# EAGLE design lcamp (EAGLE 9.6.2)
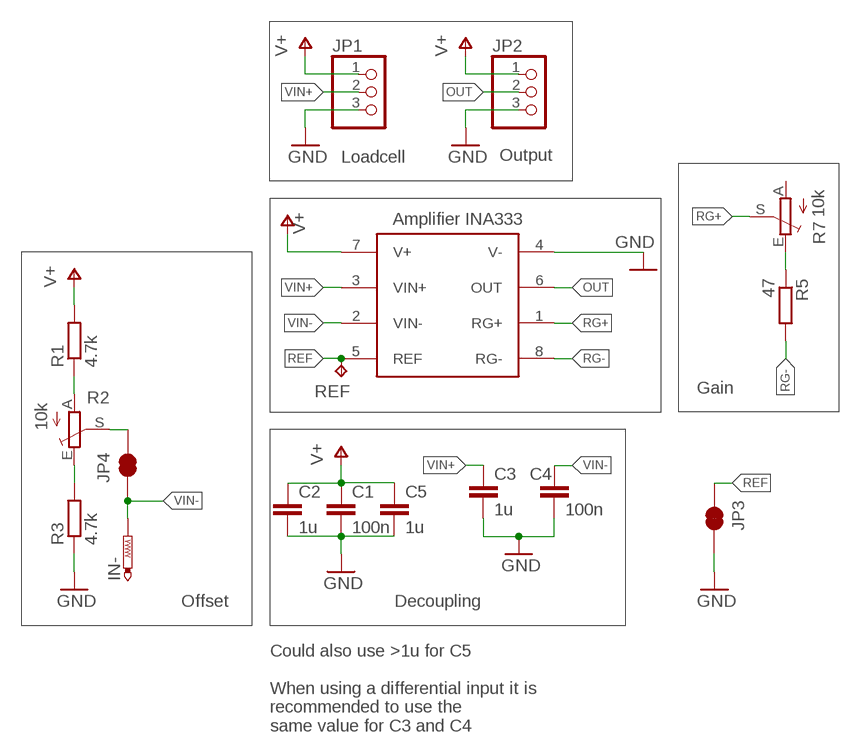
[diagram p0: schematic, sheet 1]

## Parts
C1  100n  C-EUC0603  [C0603]
C2  1u  C-EUC0603  [C0603]
C3  1u  C-EUC0603  [C0603]
C4  100n  C-EUC0603  [C0603]
C5  1u  C-EUC0603  [C0603]
IN-  PTR1PAD1-13  [P1-13]
JP1  PINHD-1X3  [1X03]
JP2  PINHD-1X3  [1X03]
JP3  JUMPER-SMT_2_NC_TRACE_SILK  [SMT-JUMPER_2_NC_TRACE_SILK]
JP4  JUMPER-SMT_2_NC_TRACE_SILK  [SMT-JUMPER_2_NC_TRACE_SILK]
R1  4.7k  R-EU_R0603  [R0603]
R2  10k  TRIM_EU-RJ9W  [RJ9W]
R3  4.7k  R-EU_R0603  [R0603]
R5  47  R-EU_R0603  [R0603]
R7  10k  TRIM_EU-RJ9W  [RJ9W]
REF  TPB1,27  [B1,27]
U1  INA333MSOP8  [MSOP8]

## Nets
GND: C1.2 C2.2 C3.2 C4.2 C5.2 JP1.3 JP2.3 JP3.2 R3.1 U1.4(V-)
N$1: R5.1 R7.E
N$2: R1.1 R2.A
N$3: R2.E R3.2
N$4: JP4.2 R2.S
OUT: JP2.2 U1.6(OUT)
REF: JP3.1 REF.TP U1.5(REF)
RG+: R7.S U1.1(RG+)
RG-: R5.2 U1.8(RG-)
V+: C1.1 C2.1 C5.1 JP1.1 JP2.1 R1.2 U1.7(V+)
VIN+: C3.1 JP1.2 U1.3(VIN+)
VIN-: C4.1 IN-.TP JP4.1 U1.2(VIN-)
Unconnected: R7.A

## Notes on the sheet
- Loadcell | Output
- Amplifier INA333
- Gain
- Offset | Decoupling
- Could also use >1u for C5
  
  When using a differential input it is
  recommended to use the 
  same value for C3 and C4

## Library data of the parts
C1-C5 = resistor:C-EU: CAPACITOR, European symbol
IN- = testpad:PTR1: TEST PIN
JP1 JP2 = pinhead:PINHD-1X3: PIN HEADER
JP3 JP4 = SparkFun-Jumpers:JUMPER-SMT_2_NC_TRACE: Normally closed trace jumper
R1 R3 R5 = resistor:R-EU_: RESISTOR, European symbol
R2 R7 = pot:TRIM_EU-: POTENTIOMETER
REF = testpad:TP: Test pad
U1 = lcamp:INA333

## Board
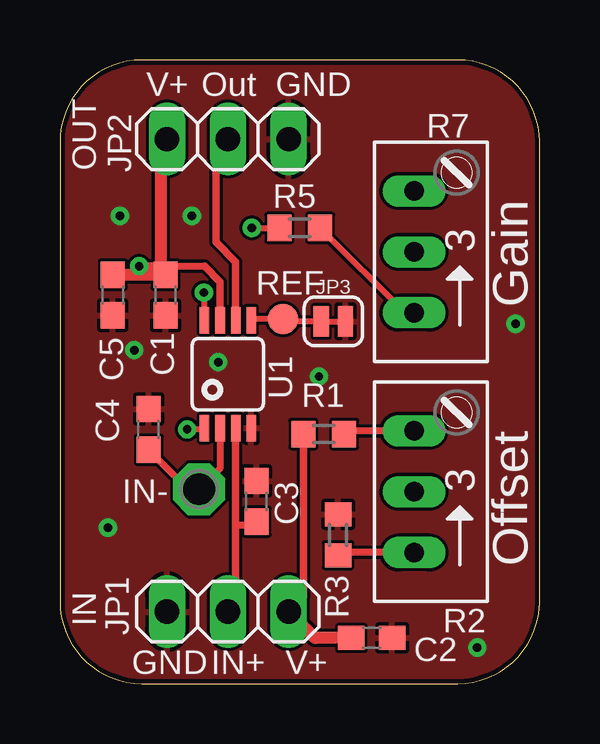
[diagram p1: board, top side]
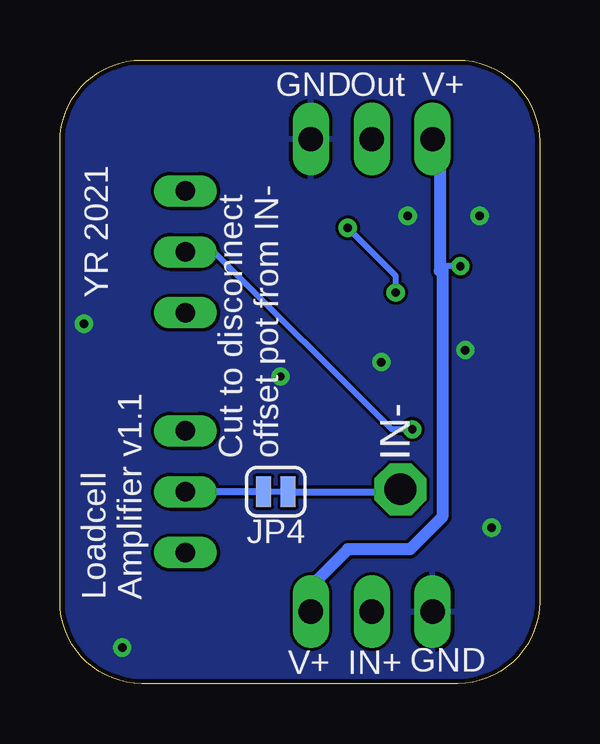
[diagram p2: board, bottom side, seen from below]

Size 20 x 26 mm. Coordinates in mm from the lower left corner, seen from the top.
Outline: 0,22.59 0,3.41 arc90 3.41,0 16.59,0 arc90 20,3.41 20,22.59 arc90 16.59,26 3.41,26 arc90 0,22.59
Copper layers (1*16): Top 0.035mm / dielectric 1.5mm / Bottom 0.035mm
Design rules "jlcpcb": minimum track width 5mil, minimum drill 0.3mm, track to track 5mil, track to pad 5mil, pad to pad 5mil, via to via 5mil, smd to smd 5mil, copper to edge 0.2mm, drill to drill 8mil, minimum pad ring 10mil, minimum via ring 8mil, stop-mask expansion 4mil, vias tented up to drill 0mil, thermal gap 6mil

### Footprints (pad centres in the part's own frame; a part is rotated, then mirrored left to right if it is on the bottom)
C0603 = smd 1.1 x 1: 1 -0.85,0; 2 0.85,0
P1-13 = drill 1.321 pad 2.159 octagon: TP 0,0
1X03 = drill 1.016 long: 1 -2.54,0; 2 0,0; 3 2.54,0
SMT-JUMPER_2_NC_TRACE_SILK = smd 0.635 x 1.27: 1 -0.508,0; 2 0.508,0
R0603 = smd 1 x 1.1: 1 -0.85,0; 2 0.85,0
RJ9W = drill 0.813 long: A 2.54,0.635; E -2.54,0.635; S 0,0.635
B1,27 = smd 1.27 x 1.27: TP 0,0
MSOP8 = smd 0.4 x 1.1: 1 -0.975,-2.25; 2 -0.325,-2.25; 3 0.325,-2.25; 4 0.975,-2.25; 5 0.975,2.25; 6 0.325,2.25; 7 -0.325,2.25; 8 -0.975,2.25

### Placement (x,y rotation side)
C1  4.4,16.2 270 top
C2  13,1.9 0 top
C3  8.2,7.6 90 top
C4  3.7,10.6 90 top
C5  2.2,16.2 270 top
IN-  5.8,8.1 0 top
JP1  7,3 180 top
JP2  7,22.7 0 top
JP3  11.4,15.1 0 top
JP4  11,8 180 bottom
R1  11,10.4 180 top
R2  15.4,8 90 top
R3  11.6,6.2 270 top
R5  10,19 180 top
R7  15.4,18 90 top
REF  9.3,15.2 0 top
U1  7,12.9 0 top

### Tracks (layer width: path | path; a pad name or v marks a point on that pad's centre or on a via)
GND  (via drill 0.35)
  other vias: 10.8,12.8 2,6.5 2.5,19.5 5.5,19.5 3.1,13.9 17.4,1.5 19,15 6.6,13.4
  pour Top: 0,27 0,-1 20,-1 20,27
  pour Bottom: 20,27 -1,27 -1,-1 20,-1
N$1
  Top 0.254: R5.1 14.39,15.46 R7.E
N$2
  Top 0.3: R2.A 11.99,10.54 R1.1
N$3
  Top 0.3: R2.E 11.71,5.46 R3.2
N$4
  Bottom 0.3: JP4.2 R2.S
OUT
  Top 0.305: U1.6 7.33,17.57 6.5,18.4 6.5,22.2 JP2.2
REF
  Top 0.254: REF.TP 8.03,15.2 U1.5 | REF.TP 9.73,15.2 | JP3.1 9.4,15.1 REF.TP
RG+  (via drill 0.35)
  Top 0.254: U1.1 6.03,10.6 v5.3,10.6
  Bottom 0.254: R7.S 13.56,18 6.17,10.6 v5.3,10.6
RG-  (via drill 0.35)
  Top 0.254: U1.8 6.03,16.27 v6,16.3 | v8,19 R5.2
  Bottom 0.254: v6,16.3 6,17 v8,19
V+  (via drill 0.35)
  Top 0.254: C1.1 4.4,17.4 | v3.3,17.4 3.4,17.3
  Top 0.3: 6.03,17.4 4.75,17.4 C1.1 4.2,17.25 4.2,17.45
  Top 0.305: R1.2 10.15,3.61 JP1.1 | U1.7 6.67,16.75 6.03,17.4 | 4.2,17.45 4.2,18.95
  Top 0.508: JP2.1 4.2,22.44 4.2,18.95 4.2,17.3 3.4,17.3 | C2.1 10.64,1.9 JP1.1 | C5.1 C1.1
  Bottom 0.254: 4.06,17.3 3.96,17.4 v3.3,17.4
  Bottom 0.508: JP2.1 4.16,22.4 4.16,17.2 4.06,17.3 4.06,6.94 5.4,5.6 8,5.6 9.54,4.06 JP1.1
VIN+
  Top 0.254: 7.33,3.33 JP1.2
  Top 0.3: C3.1 8.05,6.6 7.33,6.6
  Top 0.305: U1.3 7.33,6.6 7.33,3.33
VIN-
  Top 0.3: U1.2 6.67,8.97 IN-.TP 5.35,8.1 C4.1
  Bottom 0.3: IN-.TP 5.9,8 JP4.1

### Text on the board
tPlace: V+ | Out | GND | OUT | Gain | Offset | IN | GND | IN+ | V+
bPlace: V+ | Out | GND | YR 2021 | IN- | Cut to disconnect / offset pot from IN- | Loadcell / Amplifier v1.1 | GND | IN+ | V+

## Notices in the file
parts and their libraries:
SparkFun-Jumpers: Licensing: Creative Commons ShareAlike 4.0 International - https://creativecommons.org/licenses/by-sa/4.0
